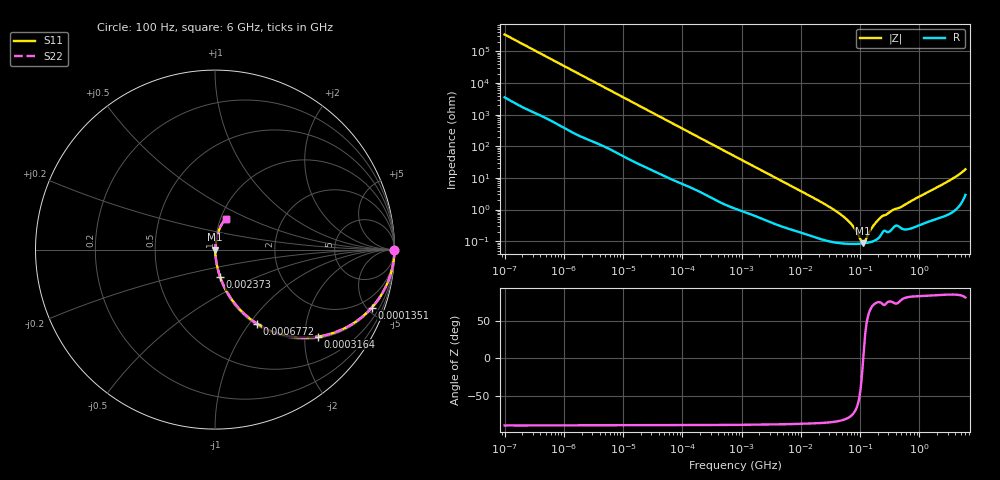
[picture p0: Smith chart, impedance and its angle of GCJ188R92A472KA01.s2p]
!Murata Part Number: GCJ188R92A472KA01
!These Parameters are Measured in Series Mode Connection
!Data Generated on Mar 13, 2026
!  o--ll--o
!Port1  Port2
!  o------o
!Operation Temp=25[degC], DC Bias Voltage=0[V]
!Freq. Start=100[Hz] Stop=6[GHz] 401[Steps]
# Hz S RI R 50
!Freq.(Hz) S11(Real) S11(Imag) S21(Real) S21(Imag) S12(Real) S12(Imag) S22(Real) S22(Imag)
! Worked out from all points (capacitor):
!   401 points, 100 Hz to 6 GHz, reference 50 ohm
!   read as one part in series: C = 4.63 nF near 109 Hz
!   lowest |Z| = 85.7 mohm at 111.6 MHz (marker M1)
!   series resonance near 113.1 MHz, so ESL is about 430 pH
!   S11 on the Smith chart (normalised r, x): 100 Hz: open; 135.1 kHz: 1.10, -5.38; 316.4 kHz: 1.05, -2.32; 677.2 kHz: 1.02, -1.09; 2.373 MHz: 1.01, -0.32; 6 GHz: 1.06, +0.37
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100  1 -0.000292  3.1e-06 0.000292  3.1e-06 0.000292  1 -0.000292
2008  0.9999 -0.00574  9.81e-05 0.00574  9.81e-05 0.00574  0.9999 -0.00574
12592  0.9983 -0.0354  0.00174 0.0354  0.00174 0.0354  0.9983 -0.0354
40335  0.9859 -0.1106  0.0141 0.1106  0.0141 0.1106  0.9859 -0.1106
135116  0.8739 -0.3226  0.1261 0.3226  0.1261 0.3226  0.8739 -0.3226
316350  0.5729 -0.4849  0.4271 0.4849  0.4271 0.4849  0.5729 -0.4849
677235  0.235 -0.4134  0.765 0.4134  0.765 0.4134  0.235 -0.4134
774597  0.1919 -0.3828  0.8081 0.3828  0.8081 0.3828  0.1919 -0.3828
2372521  0.0292 -0.1537  0.9708 0.1537  0.9708 0.1537  0.0292 -0.1537
1.555665e7  0.00203 -0.0246  0.998 0.0246  0.998 0.0246  0.00203 -0.0246
3.482834e7  0.00104 -0.0103  0.999 0.0103  0.999 0.0103  0.00104 -0.0103
5.699437e7  0.000863 -0.00522  0.9991 0.00522  0.9991 0.00522  0.000863 -0.00522
7.797396e7  0.000829 -0.00269  0.9992 0.00269  0.9992 0.00269  0.000829 -0.00269
1.020051e8  0.000839 -0.000732  0.9992 0.000732  0.9992 0.000732  0.000839 -0.000732
1.115611e8  0.000851 -9.38e-05  0.9991 9.38e-05  0.9991 9.38e-05  0.000851 -9.38e-05
1.220122e8  0.00087 0.000546  0.9991 -0.000546  0.9991 -0.000546  0.00087 0.000546
1.526266e8  0.000951 0.00219  0.999 -0.00219  0.999 -0.00219  0.000951 0.00219
1.909225e8  0.00115 0.00402  0.9989 -0.00402  0.9989 -0.00402  0.00115 0.00402
2.283698e8  0.00167 0.00563  0.9983 -0.00563  0.9983 -0.00563  0.00167 0.00563
3.124326e8  0.00207 0.0079  0.9979 -0.0079  0.9979 -0.0079  0.00207 0.0079
2.142435e9  0.00817 0.0532  0.9918 -0.0532  0.9918 -0.0532  0.00817 0.0532
6e9  0.059 0.17  0.941 -0.17  0.941 -0.17  0.059 0.17
